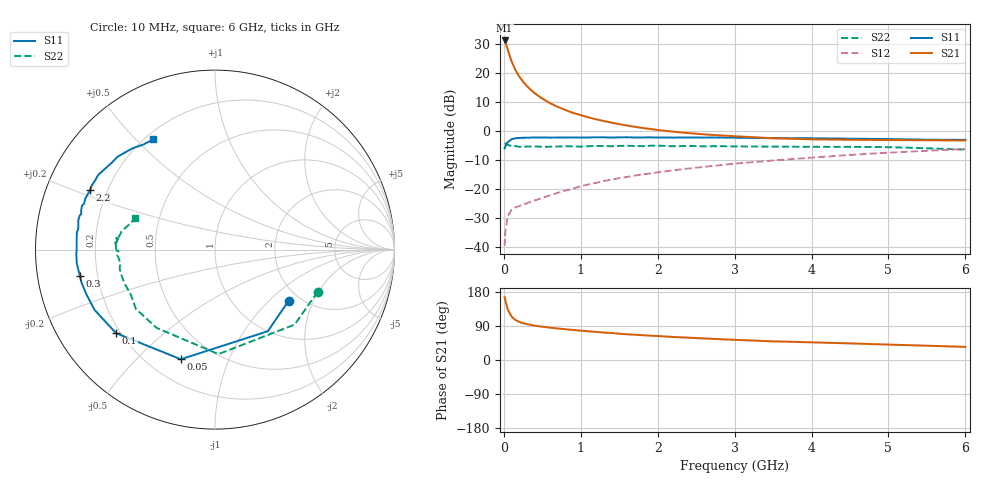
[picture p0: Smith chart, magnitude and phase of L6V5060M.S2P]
!  INFINEON TECHNOLOGIES Small Signal Semiconductors
! BFR380L3 , Si-NPN RF-Transistor in TSLP-3-1
!  Vce=0.5 V,  Ic=60 mA
! Common Emitter S-Parameters:  07. March 2005
#  GHz  S  MA  R  50
! f  S11  S21  S12  S22
! GHz  Mag  Ang  Mag  Ang  Mag  Ang  Mag  Ang
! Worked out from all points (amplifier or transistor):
!   36 points, 10 MHz to 6 GHz, reference 50 ohm
!   highest |S21| = 31.3 dB at 10 MHz (marker M1)
!   |S21| within 3 dB of that: start of sweep to 48.26 MHz
!   unconditionally stable (mu >= 1): 602 MHz to end of sweep
!   at 250 MHz: K = 0.64, MSG = 21.3 dB, |S12| = -25.4 dB
!   at 1.4 GHz: K = 1.16, MAG = 7.4 dB, |S12| = -16.8 dB
!   at 6 GHz: K = 1.07, MAG = -0.1 dB, |S12| = -6.2 dB
!   S11 on the Smith chart (normalised r, x): 10 MHz: 1.75, -1.33; 50 MHz: 0.33, -0.68; 100 MHz: 0.18, -0.36; 300 MHz: 0.13, -0.09; 2.2 GHz: 0.14, +0.22; 6 GHz: 0.23, +0.56
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0.01  0.4997 -34.7  36.9 165.8  0.0102 60.5  0.6181 -22.3
0.02  0.5417 -57.1  34.44 157.0  0.018 60.6  0.6094 -43.3
0.05  0.64 -107.3  25.68 133.4  0.0338 45.9  0.5827 -88.1
0.1  0.7216 -139.8  16.14 114.6  0.0434 35.7  0.5441 -126.7
0.15  0.7507 -153.5  11.41 105.7  0.0477 33.5  0.5509 -143.1
0.2  0.7584 -160.7  8.784 100.7  0.0504 35.3  0.5321 -151.8
0.25  0.7659 -166.0  7.142 97.2  0.0534 36.5  0.5373 -159.0
0.3  0.7668 -169.1  5.971 94.7  0.0563 39.2  0.5393 -162.0
0.4  0.7741 -174.5  4.52 90.6  0.0631 43.2  0.5422 -168.5
0.5  0.7729 -178.1  3.645 87.8  0.0698 47.2  0.534 -171.5
0.6  0.7708 179.5  3.028 85.4  0.0774 50.5  0.5353 -173.4
0.7  0.7717 177.3  2.623 83.2  0.0853 53.0  0.5402 -175.5
0.8  0.7738 174.8  2.311 81.1  0.0936 55.3  0.5462 -176.8
0.9  0.7755 172.7  2.059 79.3  0.1009 56.5  0.5433 -178.5
1.1  0.7742 169.7  1.724 75.7  0.1191 58.6  0.5475 -179.4
1.3  0.7778 165.9  1.49 72.3  0.1367 59.5  0.5489 177.6
1.6  0.7804 161.7  1.245 67.9  0.1607 60.2  0.5563 176.1
2.2  0.7708 154.6  0.976 60.8  0.209 60.4  0.5459 174.8
3.5  0.7516 139.9  0.751 49.2  0.309 56.8  0.538 171.5
4.5  0.7384 133.0  0.706 43.8  0.3862 53.1  0.5326 169.5
5.5  0.7087 124.3  0.693 37.7  0.456 47.3  0.5034 164.6
6  0.704 119.3  0.687 34.6  0.4882 44.5  0.4773 158.7
